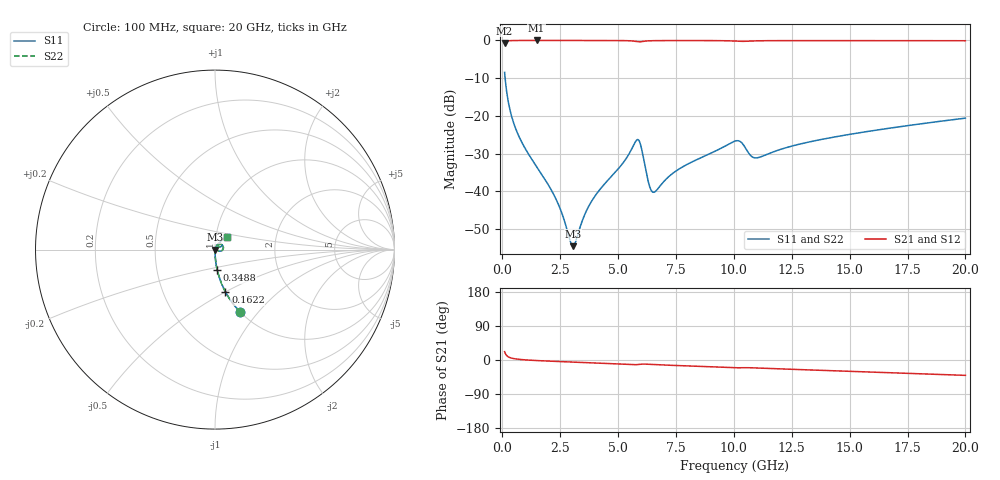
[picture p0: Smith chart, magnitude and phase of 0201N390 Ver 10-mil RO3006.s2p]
# GHz S MA R 50
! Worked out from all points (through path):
!   1601 points, 100 MHz to 20 GHz, reference 50 ohm
!   highest |S21| = -0.01 dB at 1.481 GHz (marker M1); lowest = -0.7 dB at 100 MHz (marker M2)
!   group delay of S21, straight-line fit = 5.91 ps
!   lowest |S11| = -54.5 dB at 3.048 GHz (marker M3), VSWR 1.00, Z = 50.2 - j0.0317 ohm
!   |S11| at or under -10 dB: 122 MHz to end of sweep
!   |S22| runs from -54.5 to -8.5 dB; largest |S21 - S12| = 0
!   S11 on the Smith chart (normalised r, x): 100 MHz: 1.00, -0.81; 162.2 MHz: 1.00, -0.50; 348.8 MHz: 1.00, -0.23; 20 GHz: 1.13, +0.15
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0.1  0.3766 -68.0  0.9258 21.9  0.9258 21.9  0.3766 -68.0
0.1621875  0.2428 -76.1  0.9695 13.8  0.9695 13.8  0.2428 -76.1
0.34875  0.1145 -83.7  0.9928 5.9  0.9928 5.9  0.1145 -83.7
0.74675  0.05136 -87.5  0.9978 1.6  0.9978 1.6  0.05136 -87.5
1.480563  0.02138 -88.1  0.9985 -1.4  0.9985 -1.4  0.02138 -88.1
2.33875  0.007696 -81.8  0.9983 -3.8  0.9983 -3.8  0.007696 -81.8
3.047687  0.001888 -9.6  0.998 -5.5  0.998 -5.5  0.001888 -9.6
3.420812  0.003832 51.4  0.9979 -6.3  0.9979 -6.3  0.003832 51.4
3.968062  0.008391 66.2  0.9975 -7.6  0.9975 -7.6  0.008391 66.2
5.211812  0.0238 66.2  0.9942 -10.7  0.9942 -10.7  0.0238 66.2
5.808813  0.04811 28.9  0.9631 -12.2  0.9631 -12.2  0.04811 28.9
5.982938  0.04037 -5.7  0.9596 -10.9  0.9596 -10.9  0.04037 -5.7
6.405812  0.01072 0.9  0.9894 -11.6  0.9894 -11.6  0.01072 0.9
6.542625  0.009764 22.2  0.9917 -12.1  0.9917 -12.1  0.009764 22.2
6.741625  0.01109 43.1  0.9935 -12.6  0.9935 -12.6  0.01109 43.1
7.674437  0.0202 63.0  0.9954 -14.9  0.9954 -14.9  0.0202 63.0
10.05  0.0465 46.7  0.9807 -20.4  0.9807 -20.4  0.0465 46.7
10.29875  0.04534 33.8  0.9726 -20.5  0.9726 -20.5  0.04534 33.8
10.95794  0.02782 41.0  0.9863 -21.0  0.9863 -21.0  0.02782 41.0
13.37081  0.04607 57.4  0.9937 -26.4  0.9937 -26.4  0.04607 57.4
16.69162  0.06862 52.4  0.9923 -33.5  0.9923 -33.5  0.06862 52.4
20  0.09356 46.2  0.9898 -40.5  0.9898 -40.5  0.09356 46.2
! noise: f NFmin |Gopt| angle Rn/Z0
0.1  0.000474  0.9105  0.2827  0.001164
2.301  0.003791  0.7623  4.158  0.003232
4.515  0.007116  0.7533  8.083  0.005794
6.729  0.01293  0.7934  12.06  0.01278
8.943  0.01338  0.7432  15.93  0.01026
11.14  0.02124  0.7934  19.85  0.0206
13.36  0.01617  0.6943  23.59  0.009902
15.57  0.01726  0.6723  27.32  0.009595
17.79  0.01882  0.6611  31.02  0.009894
20  0.02049  0.6539  34.67  0.01032
